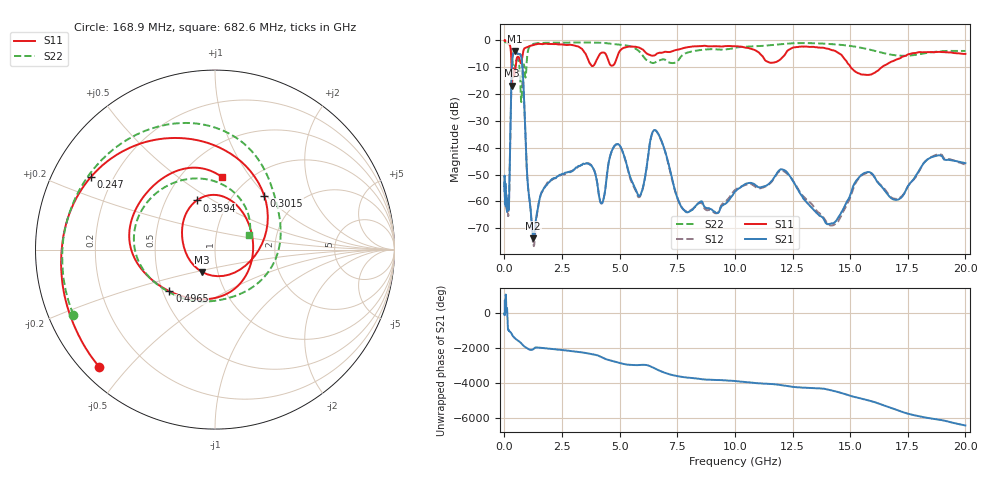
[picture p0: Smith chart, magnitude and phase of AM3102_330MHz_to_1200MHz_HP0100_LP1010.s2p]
! Date/Time: Tue, Sep 11, 2018 5:13 PM
! Network Analyzer: Agilent Technologies E8362B Rev: A.07.50.63
! Sweep from 0.010 to 20.000 GHz, 1601 Points, Sweep Type: LOG
! Power Supply: 4.950 V, 0.001 A
# Hz S DB R 50
!freq MagS11 AngS11 MagS21 AngS21 MagS12 AngS12 MagS22 AngS22
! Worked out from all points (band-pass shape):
!   1601 points, 10 MHz to 20 GHz, reference 50 ohm
!   highest |S21| = -3.89 dB at 458 MHz (marker M1); lowest = -73.7 dB at 1.248 GHz (marker M2)
!   |S21| within 3 dB of the highest: 346.2 MHz to 747.9 MHz (401.7 MHz wide, 73.4 % of centre)
!   lowest |S11| = -16.8 dB at 330 MHz (marker M3), VSWR 1.34, Z = 42.1 - j10.7 ohm
!   |S11| at or under -10 dB: 308 MHz to 487.2 MHz (179.2 MHz wide, 45.1 % of centre); 15.03 GHz to 16.37 GHz (1.348 GHz wide, 8.58 % of centre)
!   |S22| runs from -23.0 to -0.3 dB; largest |S21 - S12| = 0.012
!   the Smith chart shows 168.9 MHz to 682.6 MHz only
!   S11 on the Smith chart (normalised r, x): 168.9 MHz: 0.05, -0.42; 247 MHz: 0.12, +0.27; 301.5 MHz: 1.35, +0.97; 359.4 MHz: 0.71, +0.42; 496.5 MHz: 0.54, -0.29; 682.6 MHz: 0.77, +0.74
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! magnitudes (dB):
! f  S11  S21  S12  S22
! 10 MHz  0.0  -50.6  -50.2  -0.3
! 35.55 MHz  0.0  -57.1  -57.9  -0.5
! 126.4 MHz  -0.4  -60.7  -61.7  -1.0
! 168.9 MHz  -0.7  -61.4  -64.2  -1.2
! 247 MHz  -1.9  -40.5  -40.6  -1.9
! 301.5 MHz  -7.8  -16.3  -16.4  -3.7
! 330 MHz  -16.8  -8.8  -8.8  -6.4
! 359.4 MHz  -10.7  -6.0  -6.1  -8.5
! 447.2 MHz  -12.4  -3.9  -3.9  -10.3
! 458 MHz  -11.8  -3.9  -3.9  -9.9
! 496.5 MHz  -9.3  -4.0  -4.2  -8.3
! 682.6 MHz  -7.8  -5.1  -5.1  -13.7
! 1.248 GHz  -1.8  -73.7  -76.1  -1.3
! 1.59 GHz  -1.4  -57.1  -57.2  -0.9
! 4.23 GHz  -4.5  -60.7  -60.7  -0.9
! 4.878 GHz  -6.6  -38.6  -38.7  -1.5
! 5.652 GHz  -2.3  -54.7  -55.2  -2.9
! 6.58 GHz  -5.2  -33.6  -33.7  -8.0
! 7.92 GHz  -2.6  -64.0  -63.7  -4.6
! 12.03 GHz  -6.6  -48.0  -48.5  -1.4
! 14.21 GHz  -3.6  -68.2  -68.9  -1.4
! 20 GHz  -5.0  -45.7  -46.3  -3.9
